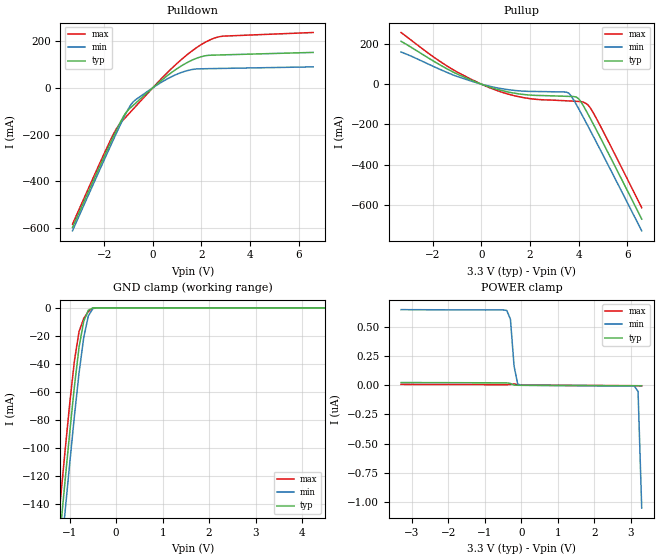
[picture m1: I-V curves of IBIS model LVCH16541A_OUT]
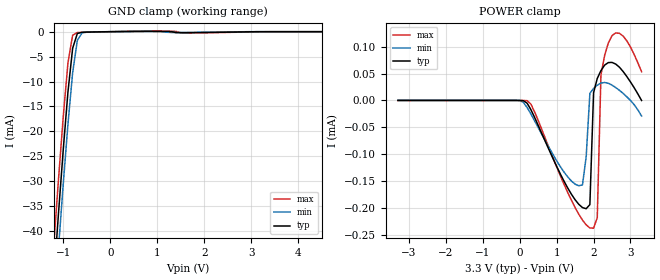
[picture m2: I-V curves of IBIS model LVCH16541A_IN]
|TEXAS INSTRUMENTS INCORPORATED
|Standard Linear and Logic Group
|IBIS Model of LVCH16541A
|16-BIT CMOS Buffer/Driver with 3-state outputs
|TSSOP 48-pin (DGG)and SSOP 48-pin (DL) Package
[IBIS Ver]   2.1
[Comment char]  |_char
[File Name]   lvch16541a.ibs
[File Rev]   1.0
[Date]   10/8/97
[Source]   File originated at Texas Instruments, Inc.
[Notes]   The following is an IBIS list for the LVCH16541A.
|   - All test data contained in this file are derived from
|   hspice(tm) simulations.
|   - File created by Ramzi Ammar, SLL Applications
|   - This file may be incomplete or may not be fully compliant
|   with the IBIS specification. It will be replaced with a
|   version that is IBIS Revision 3.2 compliant and is complete
|   and accurate.
|   Please email all questions and comments to sllibis@ti.com.
[Disclaimer] Property of Texas Instruments Incorporated.  Unauthorized
   reproduction and/or distribution is strictly prohibited.
   This product is protected under copyright law.
   Created 1997, (C) Copyright 1997, Texas Instruments Inc.,
   All Rights Reserved
   UNLESS THERE IS A SIGNED, WRITTEN AGREEMENT TO THE
   CONTRARY, TEXAS INSTRUMENTS ("TI") IS PROVIDING THE IBIS
   MODELS "AS IS" AND WITHOUT ANY WARRANTY, EXPRESSED OR
   IMPLIED.  TI assumes no liability for:
   1) the accuracy of the IBIS models provided to your
   company;
   2) the proper functioning of these IBIS models in your
   design or for any resulting applications; or
   3) infringement of patents, copyrights or intellectual
   property rights resulting from your use of these IBIS
   models.
   TI provides IBIS Models as a service to our customers.
   You and your company shall not distribute, sell or give
   these models to anyone else without prior written
   permission from TI.
   TI reserves the right to make changes to our products or
   to discontinue any semiconductor product or service
   without notice, and advises our customers to obtain the
   latest version of relevant information to verify, before
   placing orders, that the information being relied on is
   current.
   Please be aware that your receipt and use of the IBIS
   information provided shall serve as acceptance of these
   terms and conditions.  If you do not accept these terms,
   you should return or destroy the IBIS models and any
   other accompanying information immediately.
[Component]   LVCH16541A_DGG
[Manufacturer]  Texas Instruments, Inc.
[Package]
|   typ   min   max
R_pkg   0.056   0.039   0.068
L_pkg   3.390nH   3.078nH   3.995nH
C_pkg   0.520pF   0.414pF   0.668pF
[Pin]	signal_name	 model_name   R_pin   L_pin	C_pin
1   10E   NC   0.039	3.987nH	0.654pF
2   1Y1	 LVCH16541A_OUT  0.047	3.725nH	0.659pF
3   1Y2	 LVCH16541A_OUT  0.059	3.692nH	0.604pF
4   GND	 GND   0.068	3.675nH	0.606pF
5   1Y3	 LVCH16541A_OUT  0.055	3.473nH	0.547pF
6   1Y4	 LVCH16541A_OUT  0.056	3.402nH	0.497pF
7   VCC	 POWER   0.057	3.3nH   0.492pF
8   1Y5	 LVCH16541A_OUT  0.056	3.189nH	0.455pF
9   1Y6	 LVCH16541A_OUT  0.058	3.154nH	0.449pF
10   GND	 GND   0.058	3.094nH	0.436pF
11   1Y7	 LVCH16541A_OUT  0.058	3.078nH	0.424pF
12   1Y8	 LVCH16541A_OUT  0.06	3.081nH	0.414pF
13   2Y1	 LVCH16541A_OUT  0.061	3.097nH	0.416pF
14   2Y2	 LVCH16541A_OUT  0.06	3.126nH	0.427pF
15   GND	 GND   0.061	3.158nH	0.44pF
16   2Y3	 LVCH16541A_OUT  0.058	3.173nH	0.45pF
17   2Y4	 LVCH16541A_OUT  0.056	3.189nH	0.455pF
18   VCC	 POWER   0.056	3.265nH	0.49pF
19   2Y5	 LVCH16541A_OUT  0.054	3.322nH	0.492pF
20   2Y6	 LVCH16541A_OUT  0.052	3.388nH	0.544pF
21   GND	 GND   0.064	3.591nH	0.605pF
22   2Y7	 LVCH16541A_OUT  0.059	3.677nH	0.612pF
23   2Y8 	 LVCH16541A_OUT  0.046	3.678nH	0.668pF
24   2OE1	 NC   0.041	3.979nH	0.659pF
25   2OE2	 NC   0.04	3.995nH	0.658pF
26   2A8	 LVCH16541A_IN   0.046	3.69nH	0.662pF
27   2A7	 LVCH16541A_IN   0.057	3.649nH	0.602pF
28   GND	 GND   0.066	3.615nH	0.602pF
29   2A6	 LVCH16541A_IN   0.055	3.447nH	0.547pF
30   2A5	 LVCH16541A_IN   0.054	3.326nH	0.492pF
31   VCC	 POWER   0.055	3.239nH	0.488pF
32   2A4	 LVCH16541A_IN   0.056	3.183nH	0.454pF
33   2A3	 LVCH16541A_IN   0.057	3.144nH	0.447pF
34   GND	 GND   0.058	3.099nH	0.436pF
35   2A2	 LVCH16541A_IN   0.059	3.086nH	0.425pF
36   2A1	 LVCH16541A_IN   0.06	3.081nH	0.414pF
37   1A8	 LVCH16541A_IN   0.061	3.097nH	0.415pF
38   1A7	 LVCH16541A_IN   0.06	3.119nH	0.427pF
39   GND	 GND   0.06	3.144nH	0.439pF
40   1A6	 LVCH16541A_IN   0.056	3.13nH	0.446pF
41   1A5	 LVCH16541A_IN   0.057	3.208nH	0.456pF
42   VCC 	 POWER   0.056	3.247nH	0.487pF
43   1A4	 LVCH16541A_IN   0.054	3.328nH	0.491pF
44   1A3	 LVCH16541A_IN   0.053	3.413nH	0.546pF
45   GND	 GND   0.066	3.609nH	0.606pF
46   1A2	 LVCH16541A_IN   0.058	3.689nH	0.607pF
47   1A1	 LVCH16541A_IN   0.047	3.727nH	0.662pF
48   1OE2	 NC   0.04	3.978nH	0.655pF
|   Component LVCH16541A_DL
[Component]   LVCH16541A_DL
[Manufacturer]  Texas Instruments, Inc.
[Package]
|   typ	  min   max
R_pkg   0.048	  0.038	 0.053
L_pkg   6.046nH	  5.084nH   7.968nH
C_pkg   0.813pF	  0.569pF   1.157pF
[Pin]	 signal_name  model_name	R_pin   L_pin	  C_pin
1   1OE1	  NC   0.046   7.968nH	  1.017pF
2   1Y1	  LVCH16541A_OUT	0.044   7.299nH	  1.157pF
3   1Y2	  LVCH16541A_OUT	0.043   6.765nH	  1.058pF
4   GND	  GND   0.041   6.269nH	  0.933pF
5   1Y3	  LVCH16541A_OUT	0.038   5.856nH	  0.829pF
6   1Y4	  LVCH16541A_OUT	0.046   5.802nH	  0.79pF
7   VCC	  POWER   0.05   5.656nH	  0.738pF
8   1Y5	  LVCH16541A_OUT	0.053   5.5nH	  0.643pF
9   1Y6	  LVCH16541A_OUT	0.052   5.304nH	  0.606pF
10   GND	  GND   0.053   5.189nH	  0.583pF
11   1Y7	  LVCH16541A_OUT	0.051   5.084nH	  0.569pF
12   1Y8	  LVCH16541A_OUT	0.053   5.862nH	  0.833pF
13   2Y1	  LVCH16541A_OUT	0.053   5.862nH	  0.833pF
14   2Y2	  LVCH16541A_OUT	0.051   5.084nH	  0.569pF
15   GND	  GND   0.053   5.189nH	  0.583pF
16   2Y3	  LVCH16541A_OUT	0.052   5.304nH	  0.606pF
17   2Y4	  LVCH16541A_OUT	0.053   5.5nH	  0.643pF
18   VCC	  POWER   0.05   5.656nH	  0.738pF
19   2Y5	  LVCH16541A_OUT	0.046   5.802nH	  0.79pF
20   2Y6	  LVCH16541A_OUT	0.038   5.856nH	  0.829pF
21   GND	  GND   0.041   6.269nH	  0.933pF
22   2Y7	  LVCH16541A_OUT	0.043   6.765nH	  1.058pF
23   2Y8	  LVCH16541A_OUT	0.044   7.299nH	  1.157pF
24   2OE1	  NC   0.046   7.968nH	  1.017pF
25   2OE2	  NC   0.046   7.968nH	  1.017pF
26   2A8	  LVCH16541A_IN	0.044   7.299nH	  1.157pF
27   2A7	  LVCH16541A_IN	0.043   6.765nH	  1.058pF
28   GND	  GND   0.041   6.269nH	  0.933pF
29   2A6	  LVCH16541A_IN	0.038   5.856nH	  0.829pF
30   2A5	  LVCH16541A_IN	0.046   5.802nH	  0.79pF
31   VCC	  POWER   0.05   5.656nH	  0.738pF
32   2A4	  LVCH16541A_IN	0.053   5.5nH	  0.643pF
33   2A3	  LVCH16541A_IN	0.052   5.304nH	  0.606pF
34   GND	  LVCH16541A_IN	0.053   5.189nH	  0.583pF
35   2A2	  LVCH16541A_IN	0.051   5.084nH	  0.569pF
36   2A1	  LVCH16541A_IN	0.053   5.862nH	  0.833pF
37   1A8	  LVCH16541A_IN	0.053   5.862nH	  0.833pF
38   1A7	  LVCH16541A_IN	0.051   5.084nH	  0.569pF
39   GND	  GND   0.053   5.189nH	  0.583pF
40   1A6	  LVCH16541A_IN	0.052   5.304nH	  0.606pF
41   1A5	  LVCH16541A_IN	0.053   5.5nH	  0.643pF
42   VCC	  POWER   0.05   5.656nH	  0.738pF
43   1A4	  LVCH16541A_IN	0.046   5.802nH	  0.79pF
44   1A3	  LVCH16541A_IN	0.038   5.856nH	  0.829pF
45   GND	  GND   0.041   6.269nH	  0.933pF
46   1A2	  LVCH16541A_IN	0.043   6.765nH	  1.058pF
47   1A1	  LVCH16541A_IN	0.044   7.299nH	  1.157pF
48   1OE2	  NC   0.046   7.967nH	  1.017pF
| Models and submodels in the file (2): LVCH16541A_OUT (3-state), LVCH16541A_IN (Input)
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|   Model LVCH16541A_OUT
[Model]   LVCH16541A_OUT
Model_type   3-state
Polarity   Inverting
Enable   Active-Low
|   typ   min   max
C_comp   6pF   NA   NA
[Voltage range]   3.3   3.0   3.6
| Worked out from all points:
|   slope of the pulldown table from 0 to 0.495 V, typ, clamps not added: 11.3 ohm
|   slope of the pullup table from 0 to 0.495 V, typ, clamps not added: 24.5 ohm
|   GND clamp passes 1 mA (typ) near -0.56 V on its own axis
[Pullup]   | Note: Vtable = Vcc - Voutput
|   Voltage   I(typ)   I(min)   I(max)
-3.3V     212.6mA    159.2mA    256.3mA
-1.4V     75.37mA    57.61mA    89.37mA
300mV     -12.81mA   -9.33mA    -15.83mA
1.1V      -38.93mA   -27.46mA   -49.35mA
1.8V      -52.23mA   -35.29mA   -68.33mA
3.6V      -60.94mA   -45.07mA   -83.49mA
3.9V      -63.84mA   -99.17mA   -85.29mA
4V        -72.01mA   -120.8mA   -85.9mA
4.3V      -129.1mA   -188.1mA   -95.37mA
4.5V      -173.8mA   -234.1mA   -120.8mA
5.1V      -313.1mA   -374mA     -254.7mA
6.6V      -670mA     -728.7mA   -613.7mA
[Pulldown]
|   Voltage   I(typ)   I(min)   I(max)
-3.3V     -598.8mA   -613.3mA   -584.7mA
-1.6V     -205.2mA   -218.5mA   -195.5mA
-1.2V     -121.8mA   -130mA     -136.1mA
-1V       -94.08mA   -89.51mA   -113.3mA
-800mV    -74.65mA   -59.59mA   -90.59mA
0V        -3.3nA     -4.333nA   -4.892nA
700mV     60.14mA    44.1mA     75.42mA
1.4V      107.6mA    73.47mA    140.9mA
2V        133.7mA    81.92mA    185.9mA
2.5V      140.5mA    82.84mA    212.1mA
2.9V      141.6mA    83.57mA    222mA
6.6V      152.1mA    90.12mA    237.6mA
[GND_Clamp]
|   Voltage   I(typ)   I(min)   I(max)
-3.3V     -940.2mA   -961.3mA   -919.6mA
-1.3V     -194.1mA   -216.5mA   -172.5mA
-1.2V     -158.3mA   -180.6mA   -136.7mA
-1.1V     -123.1mA   -145.3mA   -101.7mA
-1V       -88.75mA   -110.7mA   -68.15mA
-900mV    -56.29mA   -77.35mA   -37.92mA
-800mV    -28.19mA   -46.53mA   -16.93mA
-700mV    -9.72mA    -21.45mA   -7.687mA
-600mV    -1.738mA   -5.758mA   -2.711mA
-500mV    -27.59uA   -482.5uA   -163uA
-300mV    -50.39nA   -1.054uA   -532.7nA
6.6V      24.57nA    651.5nA    8.554nA
[POWER_Clamp]   | Note: Vtable = Vcc - Voutput
|   Voltage   I(typ)   I(min)   I(max)
-3.3V     24.57nA    651.1nA    8.839nA
-400mV    21.8nA     644.1nA    6.218nA
-300mV    16.84nA    568.1nA    7.233nA
-200mV    2.935nA    165.5nA    13.44nA
-100mV    1.179nA    10.72nA    5.969nA
0V        999.5pA    1.191nA    2.984nA
3.1V      -3.034nA   -6.662nA   -2.564nA
3.2V      -3.164nA   -52.78nA   -2.715nA
3.3V      -3.3nA     -1.054uA   -2.87nA
[Ramp]
| variable   typ   min   max
dV/dt_r   1.2530E+00/4.1644E-10  9.6430E-01/5.5227E-10  1.4929E+00/3.6070E-10
dV/dt_f   1.6305E+00/5.5540E-10  1.3822E+00/8.9842E-10  1.8432E+00/4.0339E-10
|   Model LVCH16541A_IN
[Model]   LVCH16541A_IN
Model_type   Input
Polarity   Inverting
Vinl = 0.8V
Vinh = 2.0V
|variable   typ   min   max
C_comp   5pF   NA   NA
[Voltage Range]   3.3   3.0   3.6
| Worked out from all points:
|   GND clamp passes 1 mA (typ) near -0.72 V on its own axis
[POWER_Clamp]   | Note: Vtable = Vcc - Voutput
|   Voltage   I(typ)   I(min)   I(max)
-3.3V     16.94nA    434.2nA    3.767nA
200mV     -5.059uA   -13.02uA   -401nA
1.5V      -184.9uA   -155.8uA   -199.5uA
1.7V      -199.5uA   -157uA     -222.7uA
1.8V      -201.5uA   -104.7uA   -231.6uA
1.9V      -194uA     13.24uA    -237.4uA
2V        14.37uA    22.39uA    -237.8uA
2.1V      40.95uA    28.47uA    -218.3uA
2.2V      55.67uA    32.48uA    47.56uA
2.4V      70.58uA    32.05uA    107.1uA
2.8V      53.94uA    13.17uA    119.9uA
3.3V      -850.1pA   -28.98uA   53.62uA
[GND_Clamp]
|   Voltage   I(typ)   I(min)   I(max)
-3.3V     -345.1mA   -351.3mA   -339mA
-1.2V     -49.5mA    -56.5mA    -42.68mA
-1.1V     -36.36mA   -43.34mA   -29.55mA
-1V       -23.72mA   -30.59mA   -17.07mA
-900mV    -12.13mA   -18.59mA   -6.283mA
-800mV    -3.334mA   -8.208mA   -707.6uA
-700mV    -361.5uA   -1.751mA   -177.2uA
-600mV    -115.7uA   -247.2uA   -138.9uA
-400mV    -62.61uA   -45.49uA   -87.06uA
900mV     70.58uA    28.47uA    125.1uA
1.6V      -199.5uA   -150uA     -237.8uA
6.6V      16.94nA    434.4nA    3.558nA
